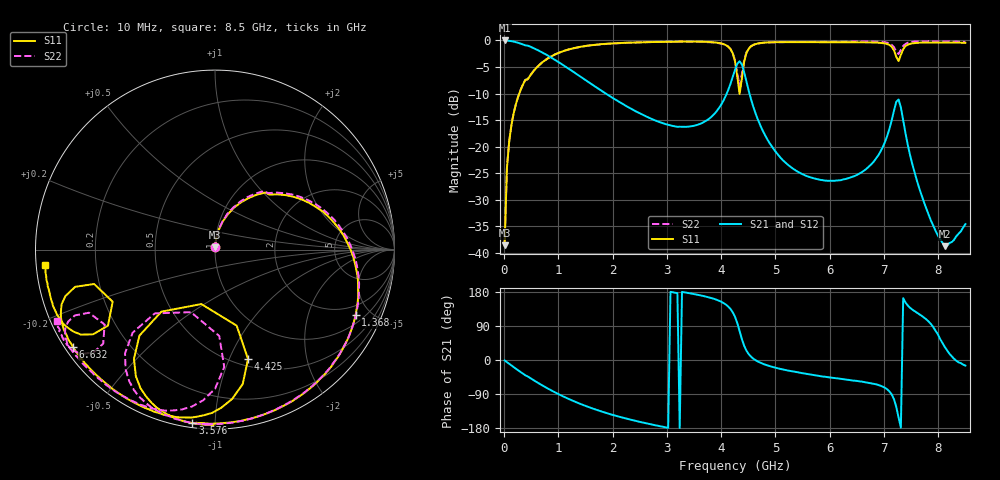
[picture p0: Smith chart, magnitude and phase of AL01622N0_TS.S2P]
!AVX CORPORATION
!PART NUMBER AL01622N0_TS
!DESCRIPTION: AIR CORE INDUCTOR, 22nH, 4 TURNS
!Agilent Technologies,E5071C,MY46102230,A.09.54
!Date: Mon Sep 03 16:34:36 2012
!Data & Calibration Information:
!Freq	S11:SOLT2(ON)	S21:SOLT2(ON)	S12:SOLT2(ON)	S22:SOLT2(ON)
# Hz S dB R 50
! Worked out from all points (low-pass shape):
!   201 points, 10 MHz to 8.5 GHz, reference 50 ohm
!   highest |S21| = -0.01 dB at 10 MHz (marker M1); lowest = -38.7 dB at 8.118 GHz (marker M2)
!   |S21| within 3 dB of the highest: start of sweep to 831.7 MHz
!   lowest |S11| = -38.6 dB at 10 MHz (marker M3), VSWR 1.02, Z = 50 + j1.18 ohm
!   |S11| at or under -10 dB: start of sweep to 280.5 MHz; 4.33868 GHz to 4.341248 GHz (2.568 MHz wide, 0.0592 % of centre)
!   |S22| runs from -38.5 to -0.2 dB; largest |S21 - S12| = 0.018
!   S11 on the Smith chart (normalised r, x): 10 MHz: 1.00, +0.02; 1.368 GHz: 1.40, -4.04; 3.576 GHz: 0.02, -0.88; 4.425 GHz: 0.57, -1.18; 6.632 GHz: 0.02, -0.31; 8.5 GHz: 0.03, -0.05
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1e7  -38.56 87.5  -0.01 -1.1  -0.14 -0.6  -38.47 85.5
5.245e7  -24.04 84.0  -0.03 -5.7  0.01 -5.8  -23.96 84.2
9.49e7  -18.96 79.2  -0.07 -10.2  -0.06 -10.2  -18.93 79.5
3.0715e8  -9.26 56.8  -0.60 -32.0  -0.58 -32.1  -9.23 58.1
7.3165e8  -3.91 19.4  -2.42 -69.2  -2.41 -69.3  -3.89 20.9
1.3684e9  -1.27 -25.1  -6.55 -113.7  -6.54 -113.8  -1.29 -23.8
1.4533e9  -1.11 -29.9  -7.13 -118.6  -7.13 -118.6  -1.14 -28.8
2.85415e9  -0.29 -86.1  -15.33 -174.1  -15.33 -174.2  -0.28 -85.0
3.5758e9  -0.22 -97.4  -15.84 171.9  -15.84 171.8  -0.24 -100.1
4.04275e9  -0.68 -112.4  -11.31 150.5  -11.31 150.4  -0.71 -117.4
4.255e9  -3.91 -131.3  -5.54 114.0  -5.54 114.0  -3.73 -134.8
4.3399e9  -10.09 -104.1  -3.92 76.5  -3.91 76.5  -8.56 -111.0
4.4248e9  -3.92 -73.2  -6.01 37.1  -6.01 37.1  -3.66 -85.5
4.55215e9  -1.09 -87.7  -11.14 8.4  -11.13 8.4  -1.07 -98.4
4.89175e9  -0.36 -104.4  -19.31 -16.0  -19.30 -16.0  -0.38 -114.8
5.6983e9  -0.33 -124.7  -25.92 -39.7  -25.92 -39.5  -0.29 -132.8
6.6322e9  -0.35 -145.6  -24.49 -58.1  -24.54 -58.0  -0.22 -144.9
7.09915e9  -0.85 -160.4  -16.68 -82.7  -16.68 -82.7  -0.55 -152.5
7.26895e9  -3.88 -153.0  -11.11 -151.8  -11.12 -151.8  -2.58 -145.8
7.651e9  -0.43 -157.7  -27.86 120.7  -27.90 120.5  -0.19 -146.9
8.11795e9  -0.41 -167.6  -38.71 34.9  -38.61 32.9  -0.20 -151.5
8.5e9  -0.46 -174.7  -34.56 -14.7  -34.59 -15.1  -0.28 -155.8
